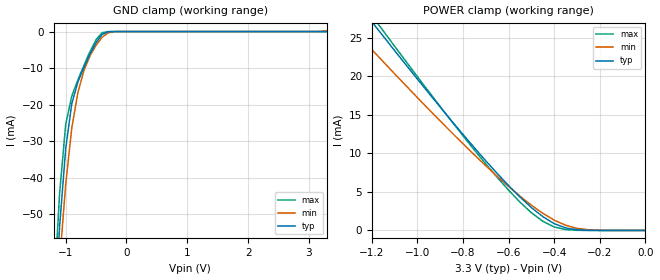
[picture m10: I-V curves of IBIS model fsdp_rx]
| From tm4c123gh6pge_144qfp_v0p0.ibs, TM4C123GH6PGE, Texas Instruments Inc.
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|   Model fsdp_rx
[Model]		fsdp_rx
Model_type	Input
C_comp   7.0000pF   7.0000pF   7.0000pF
Vinl= 1.6
Vinh= 1.7
[Temperature Range]	  27.0000   0.1250k   -40.0000
[Voltage Range]   3.3V   3.0V   3.6V
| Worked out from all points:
|   GND clamp passes 1 mA (typ) near -0.41 V on its own axis
|   POWER clamp passes 1 mA (typ) near -0.41 V on its own axis
[GND_clamp]
|Voltage	  I(typ)   I(min)   I(max)
-3.3V     -782mA     -691.8mA   -849.7mA
-1.2V     -81.21mA   -87.89mA   -73.74mA
-1.1V     -53.46mA   -63.22mA   -44.36mA
-1V       -32.12mA   -41.94mA   -25.46mA
-900mV    -19.78mA   -26.42mA   -17.7mA
-800mV    -13.86mA   -16.76mA   -13.31mA
-700mV    -9.821mA   -10.67mA   -9.261mA
-600mV    -6.194mA   -6.67mA    -5.473mA
-500mV    -3.012mA   -3.762mA   -2.229mA
-400mV    -781.4uA   -1.558mA   -310.6uA
-200mV    -1.921uA   -32.16uA   -238.5nA
3.3V      198.9nA    275.2uA    240.3nA
[POWER_clamp]
|Voltage	  I(typ)   I(min)   I(max)
-3.3V     128.2mA    118.7mA    139.8mA
-1.3V     30.83mA    26.64mA    31.9mA
-1.25V    28.94mA    25.04mA    29.88mA
-1.2V     27.06mA    23.45mA    27.87mA
-1.15V    25.18mA    21.88mA    25.87mA
-750mV    10.71mA    9.793mA    10.42mA
-600mV    5.81mA     5.697mA    5.218mA
-500mV    2.966mA    3.271mA    2.299mA
-400mV    885uA      1.333mA    454.5uA
-350mV    328.3uA    673uA      118.8uA
-250mV    20.25uA    94.06uA    3.223uA
0V        198.9nA    574.7nA    247.2nA
